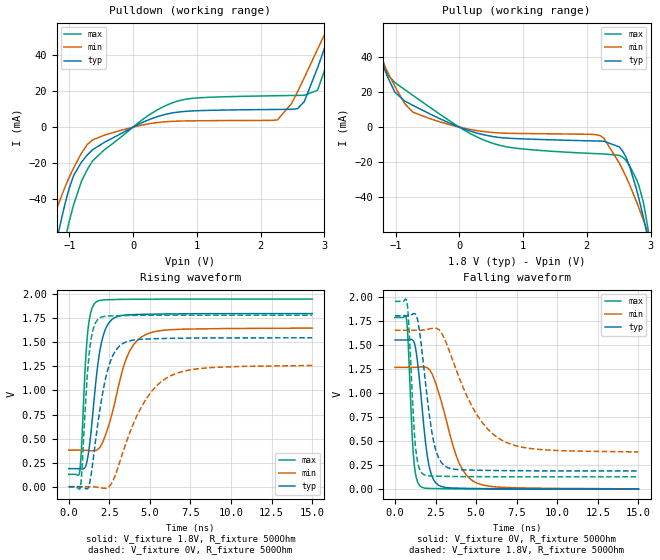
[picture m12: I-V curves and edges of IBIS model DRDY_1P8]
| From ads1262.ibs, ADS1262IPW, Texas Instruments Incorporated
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|   Model DRDY_1P8
[Model]   DRDY_1P8
Model_type   Output
Polarity   Non-Inverting
Enable   Active-Low
Vmeas = 0.9
Vref = 1.8
Cref = 15pF
Rref = 500
|   typ   min   max
|   (slow PVT)   (nom PVT)   (fast PVT)
C_comp   0.308p   0.264p   0.323p
|C_comp (ON state)   0.308p   0.269p   0.326p
|C_comp (OFF state)   0.308p   0.264p   0.323p
| Where   nom PVT is  Nominal Process, 1.8V, 27C
|   Fast PVT is Strong Process, 1.65V, -40C
|   Slow PVT is Weak Process, 1.95V, 125C
[Voltage Range]   1.8   1.65   1.95
[Temperature Range]   27   125   -40
[Pullup Reference]   1.8   1.65   1.95
[Pulldown Reference]   -0   -0   -0
[Power Clamp Reference]   1.8   1.65   1.95
[GND Clamp Reference]   -0   -0   -0
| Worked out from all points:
|   slope of the pulldown table from 0 to 0.27 V, typ, clamps not added: 61.1 ohm
|   slope of the pullup table from 0 to 0.27 V, typ, clamps not added: 82.1 ohm
|   falling waveform, V_fixture 0V, R_fixture 500Ohm: 20-80 % time 580ps typ, 1.33ns min, 297ps max; typ from 1.55 V to 0.001 V
|   rising waveform, V_fixture 1.8V, R_fixture 500Ohm: 20-80 % time 655ps typ, 1.25ns min, 347ps max; typ from 0.188 V to 1.8 V
|   rising waveform, V_fixture 0V, R_fixture 500Ohm: 20-80 % time 917ps typ, 2.06ns min, 416ps max; typ from 0 V to 1.55 V
|   falling waveform, V_fixture 1.8V, R_fixture 500Ohm: 20-80 % time 730ps typ, 2.21ns min, 348ps max; typ from 1.8 V to 0.189 V
[Pulldown]
|   Voltage   I(typ)   I(min)   I(max)
-1.8V     -174.4mA   -112.2mA   -255.8mA
-1.319V   -83.65mA   -57.54mA   -122.7mA
-1.163V   -57.14mA   -41.97mA   -82.75mA
-1.012V   -35.21mA   -28.64mA   -53.87mA
-930.6mV  -26.73mA   -22.53mA   -42.89mA
-633.6mV  -12.51mA   -7.035mA   -18.7mA
608.4mV   7.828mA    3.211mA    13.36mA
2.266V    9.815mA    4.076mA    17.44mA
2.682V    14.05mA    27.18mA    17.67mA
3.001V    43.57mA    51.17mA    31.18mA
3.173V    60.68mA    63.45mA    53.5mA
3.595V    97.16mA    89.03mA    104.8mA
[Pullup]
|   Voltage   I(typ)   I(min)   I(max)
-1.8V     87.85mA    77.49mA    102.3mA
-1.589V   71.16mA    64.46mA    81.71mA
-1.012V   19.96mA    23.25mA    25.39mA
-725.4mV  12.35mA    8.494mA    18.02mA
543.6mV   -5.461mA   -3.116mA   -9.42mA
2.201V    -7.932mA   -4.796mA   -15.17mA
2.509V    -11.25mA   -20.46mA   -16.04mA
2.671V    -22.42mA   -32.85mA   -22.07mA
2.817V    -40.84mA   -46.08mA   -33.45mA
2.893V    -52.4mA    -53.53mA   -43.99mA
2.979V    -66.57mA   -62.44mA   -61.94mA
3.595V    -181.7mA   -134.3mA   -228.1mA
[Ramp]
R_load = 500
|   typ   min   max
dV/dt_r   0.966917/6.55081e-10   0.760692/1.25453e-09   1.09301/3.4681e-10
dV/dt_f   0.928522/5.80497e-10   0.756975/1.32568e-09   1.06962/2.97037e-10
[Falling Waveform]
V_fixture = 0V
V_fixture_min = 0V
V_fixture_max = 0V
R_fixture = 500Ohm
C_fixture = 0F
|   Time   V(typ)   V(min)   V(max)
0s        1.549V     1.265V     1.783V
717.8ps   1.549V     1.264V     1.753V
1.131ns   1.54V      1.264V     361.4mV
1.315ns   1.416V     1.266V     117.8mV
1.552ns   1.06V      1.268V     31.93mV
2.109ns   232.6mV    1.243V     7.678mV
2.849ns   27.77mV    912.6mV    4.894mV
3.947ns   10.37mV    271.9mV    2.548mV
5.093ns   6.726mV    59.93mV    1.495mV
15ns      1.148mV    2.923mV    37.55uV
[Rising Waveform]
V_fixture = 1.8V
V_fixture_min = 1.65V
V_fixture_max = 1.95V
R_fixture = 500Ohm
C_fixture = 0F
|   Time   V(typ)   V(min)   V(max)
0s        187.7mV    380.5mV    128.3mV
674.2ps   186.7mV    380.7mV    153mV
1.131ns   266.2mV    378.2mV    1.534V
1.315ns   474.7mV    375.3mV    1.779V
1.661ns   1.072V     376.9mV    1.916V
2ns       1.484V     429.5mV    1.938V
2.379ns   1.679V     593.4mV    1.943V
3.542ns   1.784V     1.329V     1.947V
4.493ns   1.791V     1.557V     1.948V
15ns      1.799V     1.648V     1.95V
[Rising Waveform]
V_fixture = 0V
V_fixture_min = 0V
V_fixture_max = 0V
R_fixture = 500Ohm
C_fixture = 0F
|   Time   V(typ)   V(min)   V(max)
0s        1.029nV    3.208nV    730.2pV
717.8ps   98.06uV    237.8uV    -6.416mV
1.131ns   -22.32mV   374.6uV    1.12V
1.315ns   57.61mV    435.5uV    1.46V
1.927ns   806.4mV    -9.996mV   1.756V
2.379ns   1.2V       -11.06mV   1.773V
3.049ns   1.449V     206.3mV    1.777V
4.493ns   1.532V     832.9mV    1.781V
5.993ns   1.541V     1.126V     1.782V
15ns      1.547V     1.26V      1.783V
[Falling Waveform]
|Gnd
V_fixture = 1.8V
V_fixture_min = 1.65V
V_fixture_max = 1.95V
R_fixture = 500Ohm
C_fixture = 0F
|   Time   V(typ)   V(min)   V(max)
0s        1.8V       1.65V      1.95V
739.6ps   1.799V     1.65V      1.937V
1.253ns   1.818V     1.649V     459.2mV
1.463ns   1.692V     1.649V     233.1mV
1.794ns   1.238V     1.653V     149mV
2.379ns   495.4mV    1.671V     135.5mV
3.249ns   223.8mV    1.479V     132.8mV
4.793ns   197.5mV    845.7mV    129.9mV
6.593ns   192.6mV    507.4mV    128.8mV
15ns      189.1mV    386.4mV    128.3mV
